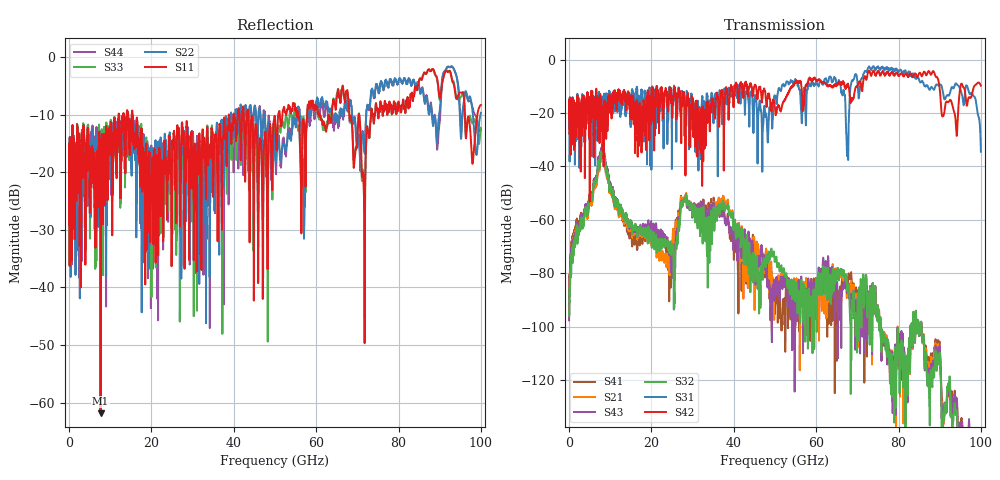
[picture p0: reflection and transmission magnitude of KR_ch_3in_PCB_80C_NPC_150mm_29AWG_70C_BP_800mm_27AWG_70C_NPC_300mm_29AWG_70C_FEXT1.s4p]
# GHz S RI R 45
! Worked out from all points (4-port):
!   4000 points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, 25 MHz to 100 GHz, reference 45 ohm
!   strongest paths, dB at 25 MHz, 25.02 GHz, 50.02 GHz, 75.03 GHz, 100 GHz:
!     S42: -20.7, -17.7, -18.0, -4.4, -9.7
!     S31: -20.6, -19.9, -13.7, -2.5, -34.5
!     S32: -94.9, -70.7, -75.0, -95.0, -155.5
!     S43: -97.7, -77.9, -85.3, -94.9, -149.9
!     S21: -88.8, -68.9, -85.0, -94.8, -156.5
!     S41: -95.3, -76.5, -90.8, -94.9, -152.5
!   lowest |S11| = -61.8 dB at 7.65 GHz (marker M1), VSWR 1.00, Z = 45 - j0.0684 ohm
!   |S11| at or under -10 dB: start of sweep to 12.07 GHz; 15.37 GHz to 38.82 GHz (23.45 GHz wide, 86.6 % of centre); 43.49 GHz to 50.81 GHz (7.32 GHz wide, 15.5 % of centre)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
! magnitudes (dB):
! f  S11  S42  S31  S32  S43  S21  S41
! 25 MHz  -16.4  -20.7  -20.6  -94.9  -97.7  -88.8  -95.3
! 7.65 GHz  -61.8  -18.4  -20.7  -36.3  -34.8  -37.3  -35.6
! 24.52 GHz  -16.8  -10.9  -11.7  -69.4  -70.5  -73.5  -76.9
! 28.05 GHz  -36.8  -17.5  -28.5  -53.2  -52.8  -53.2  -52.5
! 67.6 GHz  -5.8  -9.8  -30.2  -86.6  -85.0  -87.4  -82.1
! 78.3 GHz  -9.5  -4.9  -3.0  -111.1  -113.2  -109.7  -111.3
! 100 GHz  -8.4  -9.7  -34.5  -155.5  -149.9  -156.5  -152.5
